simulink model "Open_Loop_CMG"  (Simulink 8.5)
settings: Solver=ode45  StartTime=0.0  StopTime=10000  FixedStep=Ts*5  RelTol=1e-3
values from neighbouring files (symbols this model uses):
  Ave = [    [vehicle_flex34.m]    (also in vehicle_rigid.m)
  Bve = [    [vehicle_flex34.m]    (also in vehicle_rigid.m)
  CB2L = [cpsi, -cphi*spsi,  sphi*spsi;          0,    cphi,      -sphi;          0,    sphi*cpsi,  cphi*cpsi]/cpsi    [Rigbod_Dynam_LVLH.m]    (also in start.m = eye(3); start2.m = eye(3); start3.m = eye(3); start1.m = eye(3))
  Cve = [    [vehicle_flex34.m]    (also in vehicle_rigid.m)
  Dve = [    [vehicle_flex34.m]    (also in vehicle_rigid.m)
  ini = [wbo; atto; Hco]    [start.m]    (also in start2.m; start3.m; start1.m)
  J = [0.119416e9, -0.476e7,   -0.1216e7;     -0.476e7,     0.40408e8, -0.30121e6;     -0.1216e7,   -0.30121e6,  0.110166e9]    [start.m]    (also in start2.m; start3.m; start1.m)
  nt = 12    [start.m]    (also in start2.m; start3.m; start1.m)
  omg = 20*wo    (= 0.022)    [start.m]    (also in start2.m; start3.m; start1.m)
  wo = 0.0011    [start.m]    (also in start2.m; start3.m; start1.m)
  zeb = 0.95    [start.m]    (also in start2.m; start3.m; start1.m)
undefined symbols (not defined in the file or in its folder): Rigbod_Dynam_LVLH

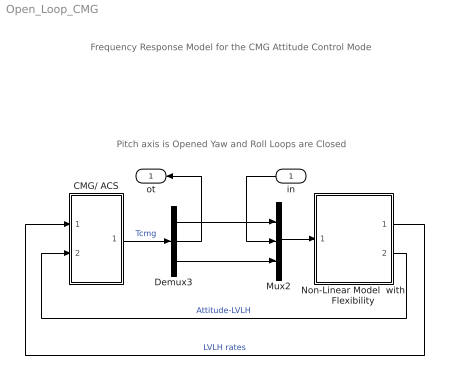
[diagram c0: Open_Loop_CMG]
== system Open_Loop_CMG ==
  note: Frequency Response Model for the CMG Attitude Control Mode
  note: Pitch axis is Opened Yaw and Roll Loops are Closed
  in : Inport
  CMG/ ACS : Subsystem
  Demux3 : Demux  Outputs=3
  Mux2 : Mux  Inputs=3
  Non-Linear Model  with Flexibility : Subsystem
  ot : Outport
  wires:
  Non-Linear Model  with Flexibility/1(wlv) -> CMG/ ACS/1(wl)  "LVLH rates"
  Non-Linear Model  with Flexibility/2(atti) -> CMG/ ACS/2(ater)  "Attitude-LVLH"
  CMG/ ACS/1(Tq) -> Demux3/1  "Tcmg"
  Mux2/1 -> Non-Linear Model  with Flexibility/1(Tcmg)
  Demux3/3 -> Mux2/3
  Demux3/1 -> Mux2/1
  Demux3/2 -> ot/1
  in/1 -> Mux2/2

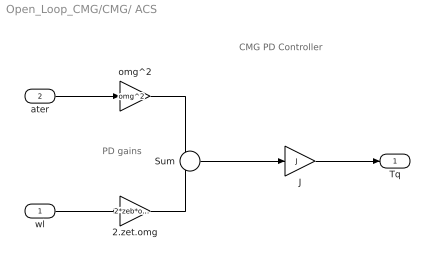
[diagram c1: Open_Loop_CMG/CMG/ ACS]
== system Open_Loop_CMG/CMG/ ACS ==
  note: CMG PD Controller
  note: PD gains
  wl : Inport
  ater : Inport  Port=2  PortDimensions=3
  2.zet.omg : Gain  Gain=2*zeb*omg
  J : Gain  Gain=J  Multiplication=Matrix(K*u)
  Sum : Sum  Inputs=--
  omg^2 : Gain  Gain=omg^2
  Tq : Outport
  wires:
  wl/1 -> 2.zet.omg/1
  Sum/1 -> J/1
  2.zet.omg/1 -> Sum/2
  ater/1 -> omg^2/1
  omg^2/1 -> Sum/1
  J/1 -> Tq/1

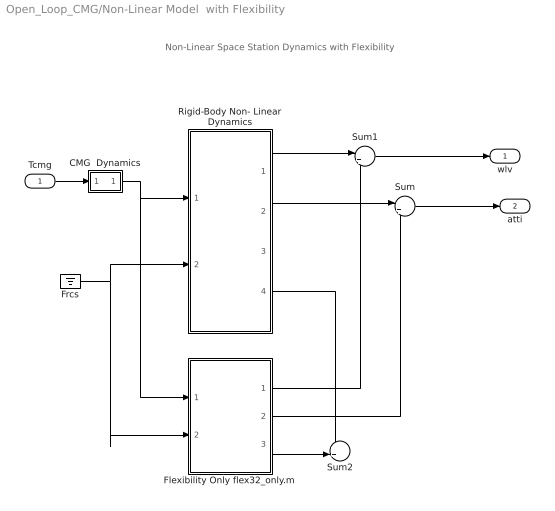
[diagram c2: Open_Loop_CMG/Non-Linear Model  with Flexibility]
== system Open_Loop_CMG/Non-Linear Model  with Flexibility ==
  note: Non-Linear Space Station Dynamics with Flexibility
  Tcmg : Inport
  CMG  Dynamics : Subsystem
  Flexibility Only flex32_only.m : Subsystem
  Frcs : Ground
  Rigid-Body Non- Linear Dynamics : Subsystem
  Sum : Sum  Inputs=|++
  Sum1 : Sum  Inputs=|++
  Sum2 : Sum  Inputs=++|
  wlv : Outport
  atti : Outport  Port=2
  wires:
  Frcs/1 -> Rigid-Body Non- Linear Dynamics/2(Frcs), Flexibility Only flex32_only.m/2(Frcs)
  Rigid-Body Non- Linear Dynamics/2(atti-lv) -> Sum/1
  Flexibility Only flex32_only.m/2(att) -> Sum/2
  Sum/1 -> atti/1
  Sum1/1 -> wlv/1
  Tcmg/1 -> CMG  Dynamics/1(I)
  Rigid-Body Non- Linear Dynamics/1(w-lv) -> Sum1/1
  Flexibility Only flex32_only.m/1(wbf) -> Sum1/2
  Flexibility Only flex32_only.m/3(wb) -> Sum2/2
  Rigid-Body Non- Linear Dynamics/4(wb) -> Sum2/1
  CMG  Dynamics/1(O) -> Rigid-Body Non- Linear Dynamics/1(Tcmg), Flexibility Only flex32_only.m/1(Tcmg)

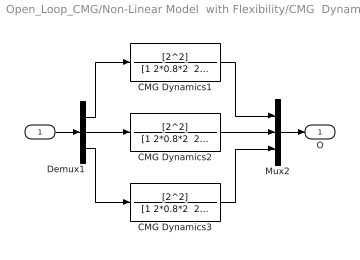
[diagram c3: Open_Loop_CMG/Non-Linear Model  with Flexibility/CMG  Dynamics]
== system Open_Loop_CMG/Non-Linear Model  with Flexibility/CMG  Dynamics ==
  I : Inport
  CMG Dynamics1 : TransferFcn  Numerator=[2^2]  Denominator="[1 2*0.8*2  2^2]"
  CMG Dynamics2 : TransferFcn  Numerator=[2^2]  Denominator="[1 2*0.8*2  2^2]"
  CMG Dynamics3 : TransferFcn  Numerator=[2^2]  Denominator="[1 2*0.8*2  2^2]"
  Demux1 : Demux  Outputs=3
  Mux2 : Mux  Inputs=3
  O : Outport
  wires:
  Mux2/1 -> O/1
  I/1 -> Demux1/1
  Demux1/3 -> CMG Dynamics3/1
  Demux1/1 -> CMG Dynamics1/1
  Demux1/2 -> CMG Dynamics2/1
  CMG Dynamics1/1 -> Mux2/1
  CMG Dynamics3/1 -> Mux2/3
  CMG Dynamics2/1 -> Mux2/2

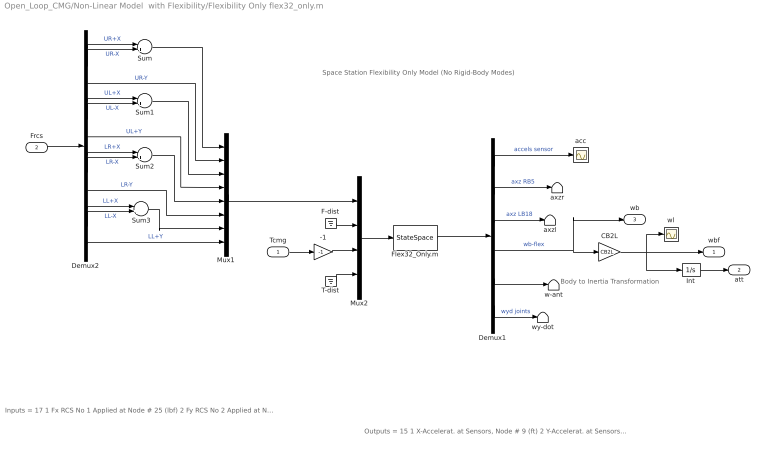
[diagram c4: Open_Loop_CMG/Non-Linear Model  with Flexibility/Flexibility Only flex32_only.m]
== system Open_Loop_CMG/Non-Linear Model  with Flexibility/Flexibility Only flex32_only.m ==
  note: Outputs = 15 1 X-Accelerat. at Sensors, Node # 9 (ft) 2 Y-Accelerat. at Sensors, Node # 9 (ft) 3 Z-Accelerat. at Sensors, Node # 9 (ft) 4 X-Accelerat. at Right Boom End, Node # 5 (ft) 5 Z-Accelerat. at Right Boom End, Node # 5 (ft) 6 X-Accelerat. at Left Boom End, Node # 18 (ft) 7 Z-Accelerat. at Left Boom End, Node # 18 (ft) 8 X-Rot. Rate at Sensors, Node # 9 (radian) 9 Y-Rot. Rate at Sensors, Node # 9 (radian) 10 Z-Rot. Rate at Sensors, Node # 9 (radian) 11 X-Rot. Rate at Antena Bot-Left, Node # 24 (radian) 12 Y-Rot. Rate at Antena Bot-Left, Node # 24 (radian) 13 Z-Rot. Rate at Antena Bot-Left, Node # 24 (radian) 14 Y-Rot.Accel. at Right Joint, Node # 7 (radian) 15 Y-Rot.Accel. at Left Joint, Node # 16 (radian)
  note: Inputs = 17 1 Fx RCS No 1 Applied at Node # 25 (lbf) 2 Fy RCS No 2 Applied at Node # 25 (lbf) 3 Fx RCS No 3 Applied at Node # 26 (lbf) 4 Fy RCS No 4 Applied at Node # 26 (lbf) 5 Fx RCS No 5 Applied at Node # 27 (lbf) 6 Fy RCS No 6 Applied at Node # 27 (lbf) 7 Fx RCS No 7 Applied at Node # 28 (lbf) 8 Fy RCS No 8 Applied at Node # 28 (lbf) 9 Fx Disturb. No 9 at Node # 21 (lbf) 10 Fy Disturb. No 10 at Node # 21 (lbf) 11 Fz Disturb. No 11 at Node # 21 (lbf) 12 Torq-x No 1 CMG Applied at Node # 10 (ft-lb) 13 Torq-y No 2 CMG Applied at Node # 10 (ft-lb) 14 Torq-z No 3 CMG Applied at Node # 10 (ft-lb) 15 Torq-x No 4 Gimbal Dist. at Node # 1 (ft-lb) 16 Torq-y No 5 Gimbal Dist. at Node # 1 (ft-lb) 17 Torq-z No 6 Gimbal Dist. at Node # 1 (ft-lb)
  note: Space Station Flexibility Only Model (No Rigid-Body Modes)
  note: Body to Inertia Transformation
  Tcmg : Inport
  Frcs : Inport  Port=2
  -1 : Gain  Gain=-1
  CB2L : Gain  Gain=CB2L  Multiplication=Matrix(K*u)
  Demux1 : Demux  Outputs=[3, 2, 2, 3, 3, 2]
  Demux2 : Demux  Outputs=12
  F-dist : Ground
  Flex32_Only.m : StateSpace  A=Ave  B=Bve  C=Cve  D=Dve  X0=0
  Int : Integrator
  Mux1 : Mux  Inputs=8
  Mux2 : Mux  Inputs=[8, 3, 3, 3]
  Sum{,1..3} (4 alike) : Sum  Inputs=|+-
  T-dist : Ground
  acc : Scope
  axzl : Terminator
  axzr : Terminator
  w-ant : Terminator
  wl : Scope
  wy-dot : Terminator
  wbf : Outport
  att : Outport  Port=2
  wb : Outport  Port=3
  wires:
  Demux1/6 -> wy-dot/1  "wyd joints"
  Demux1/5 -> w-ant/1
  T-dist/1 -> Mux2/4
  F-dist/1 -> Mux2/2
  Demux1/3 -> axzl/1  "axz LB18"
  Demux1/2 -> axzr/1  "axz RB5"
  Tcmg/1 -> -1/1
  Demux1/4 -> CB2L/1, wb/1  "wb-flex"
  Demux1/1 -> acc/1  "accels sensor"
  Flex32_Only.m/1 -> Demux1/1
  Mux2/1 -> Flex32_Only.m/1
  Mux1/1 -> Mux2/1
  Frcs/1 -> Demux2/1
  Demux2/6 -> Mux1/4  "UL+Y"
  Demux2/9 -> Mux1/6  "LR-Y"
  Demux2/12 -> Mux1/8  "LL+Y"
  Demux2/3 -> Mux1/2  "UR-Y"
  Demux2/1 -> Sum/1  "UR+X"
  Demux2/2 -> Sum/2  "UR-X"
  Sum/1 -> Mux1/1
  Demux2/4 -> Sum1/1  "UL+X"
  Demux2/5 -> Sum1/2  "UL-X"
  Sum1/1 -> Mux1/3
  Demux2/7 -> Sum2/1  "LR+X"
  Demux2/8 -> Sum2/2  "LR-X"
  Demux2/10 -> Sum3/1  "LL+X"
  Demux2/11 -> Sum3/2  "LL-X"
  Sum3/1 -> Mux1/7
  Sum2/1 -> Mux1/5
  Int/1 -> att/1
  -1/1 -> Mux2/3
  CB2L/1 -> wl/1, wbf/1, Int/1

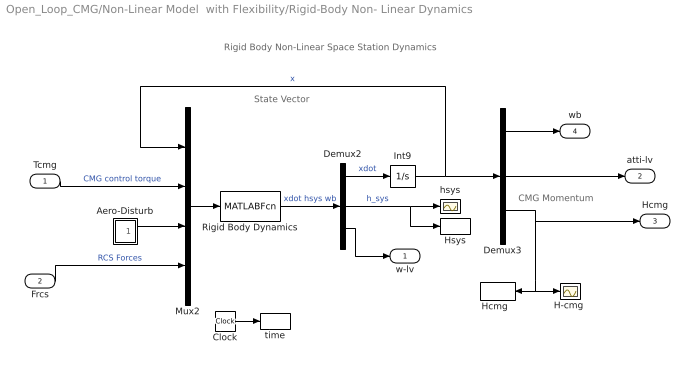
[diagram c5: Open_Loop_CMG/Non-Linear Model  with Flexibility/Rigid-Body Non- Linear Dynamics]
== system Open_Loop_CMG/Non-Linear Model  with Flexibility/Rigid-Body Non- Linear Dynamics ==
  note: CMG Momentum
  note: State Vector
  note: Rigid Body Non-Linear Space Station Dynamics
  Tcmg : Inport  PortDimensions=3
  Frcs : Inport  Port=2  PortDimensions=nt
  Aero-Disturb : Subsystem
  Clock : Clock
  Demux2 : Demux  Outputs=[9,3,3]
  Demux3 : Demux  Outputs=[3,3,3]
  "H-cmg " : Scope
  "Hcmg  " : ToWorkspace  VariableName=Hcmg  SampleTime=-1
  Hsys : ToWorkspace  VariableName=Hsys  SampleTime=-1
  Int9 : Integrator  InitialCondition=ini
  Mux2 : Mux  Inputs=[9, 3, 3, nt]
  Rigid Body Dynamics : MATLABFcn  MATLABFcn=Rigbod_Dynam_LVLH( u(1:9), u(10:12), u(13:15), u(16:15+nt) )  OutputDimensions=15
  hsys : Scope
  time : ToWorkspace  VariableName=time  SampleTime=-1
  w-lv : Outport
  atti-lv : Outport  Port=2
  Hcmg : Outport  Port=3
  wb : Outport  Port=4
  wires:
  Mux2/1 -> Rigid Body Dynamics/1
  Clock/1 -> time/1
  Frcs/1 -> Mux2/4  "RCS Forces"
  Demux3/3 -> Hcmg/1, "H-cmg "/1, "Hcmg  "/1
  Demux3/2 -> atti-lv/1
  Demux2/2 -> Hsys/1, hsys/1  "h_sys"
  Demux2/3 -> w-lv/1
  Tcmg/1 -> Mux2/2  "CMG control torque"
  Int9/1 -> Mux2/1, Demux3/1  "x"
  Demux2/1 -> Int9/1  "xdot"
  Rigid Body Dynamics/1 -> Demux2/1  "xdot hsys wb"
  Aero-Disturb/1(Td) -> Mux2/3
  Demux3/1 -> wb/1

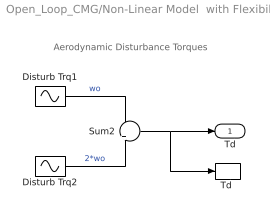
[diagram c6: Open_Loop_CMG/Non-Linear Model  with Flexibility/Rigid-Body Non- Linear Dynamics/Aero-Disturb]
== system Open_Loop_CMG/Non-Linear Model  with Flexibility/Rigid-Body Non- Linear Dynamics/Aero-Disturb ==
  note: Aerodynamic Disturbance Torques
  Disturb Trq1 : Sin  Amplitude=[1, 3, 1]  Bias="[1  8  1]"  Frequency=[wo, wo, wo]  SampleTime=0
  Disturb Trq2 : Sin  Amplitude=[1, 1, 1]*0.5  Frequency=[wo, wo, wo]*2  SampleTime=0
  Sum2 : Sum  Inputs=+|+
  "Td " : ToWorkspace  VariableName=Td  SampleTime=-1
  Td : Outport
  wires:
  Disturb Trq2/1 -> Sum2/2  "2*wo"
  Sum2/1 -> "Td "/1, Td/1
  Disturb Trq1/1 -> Sum2/1  "wo"
